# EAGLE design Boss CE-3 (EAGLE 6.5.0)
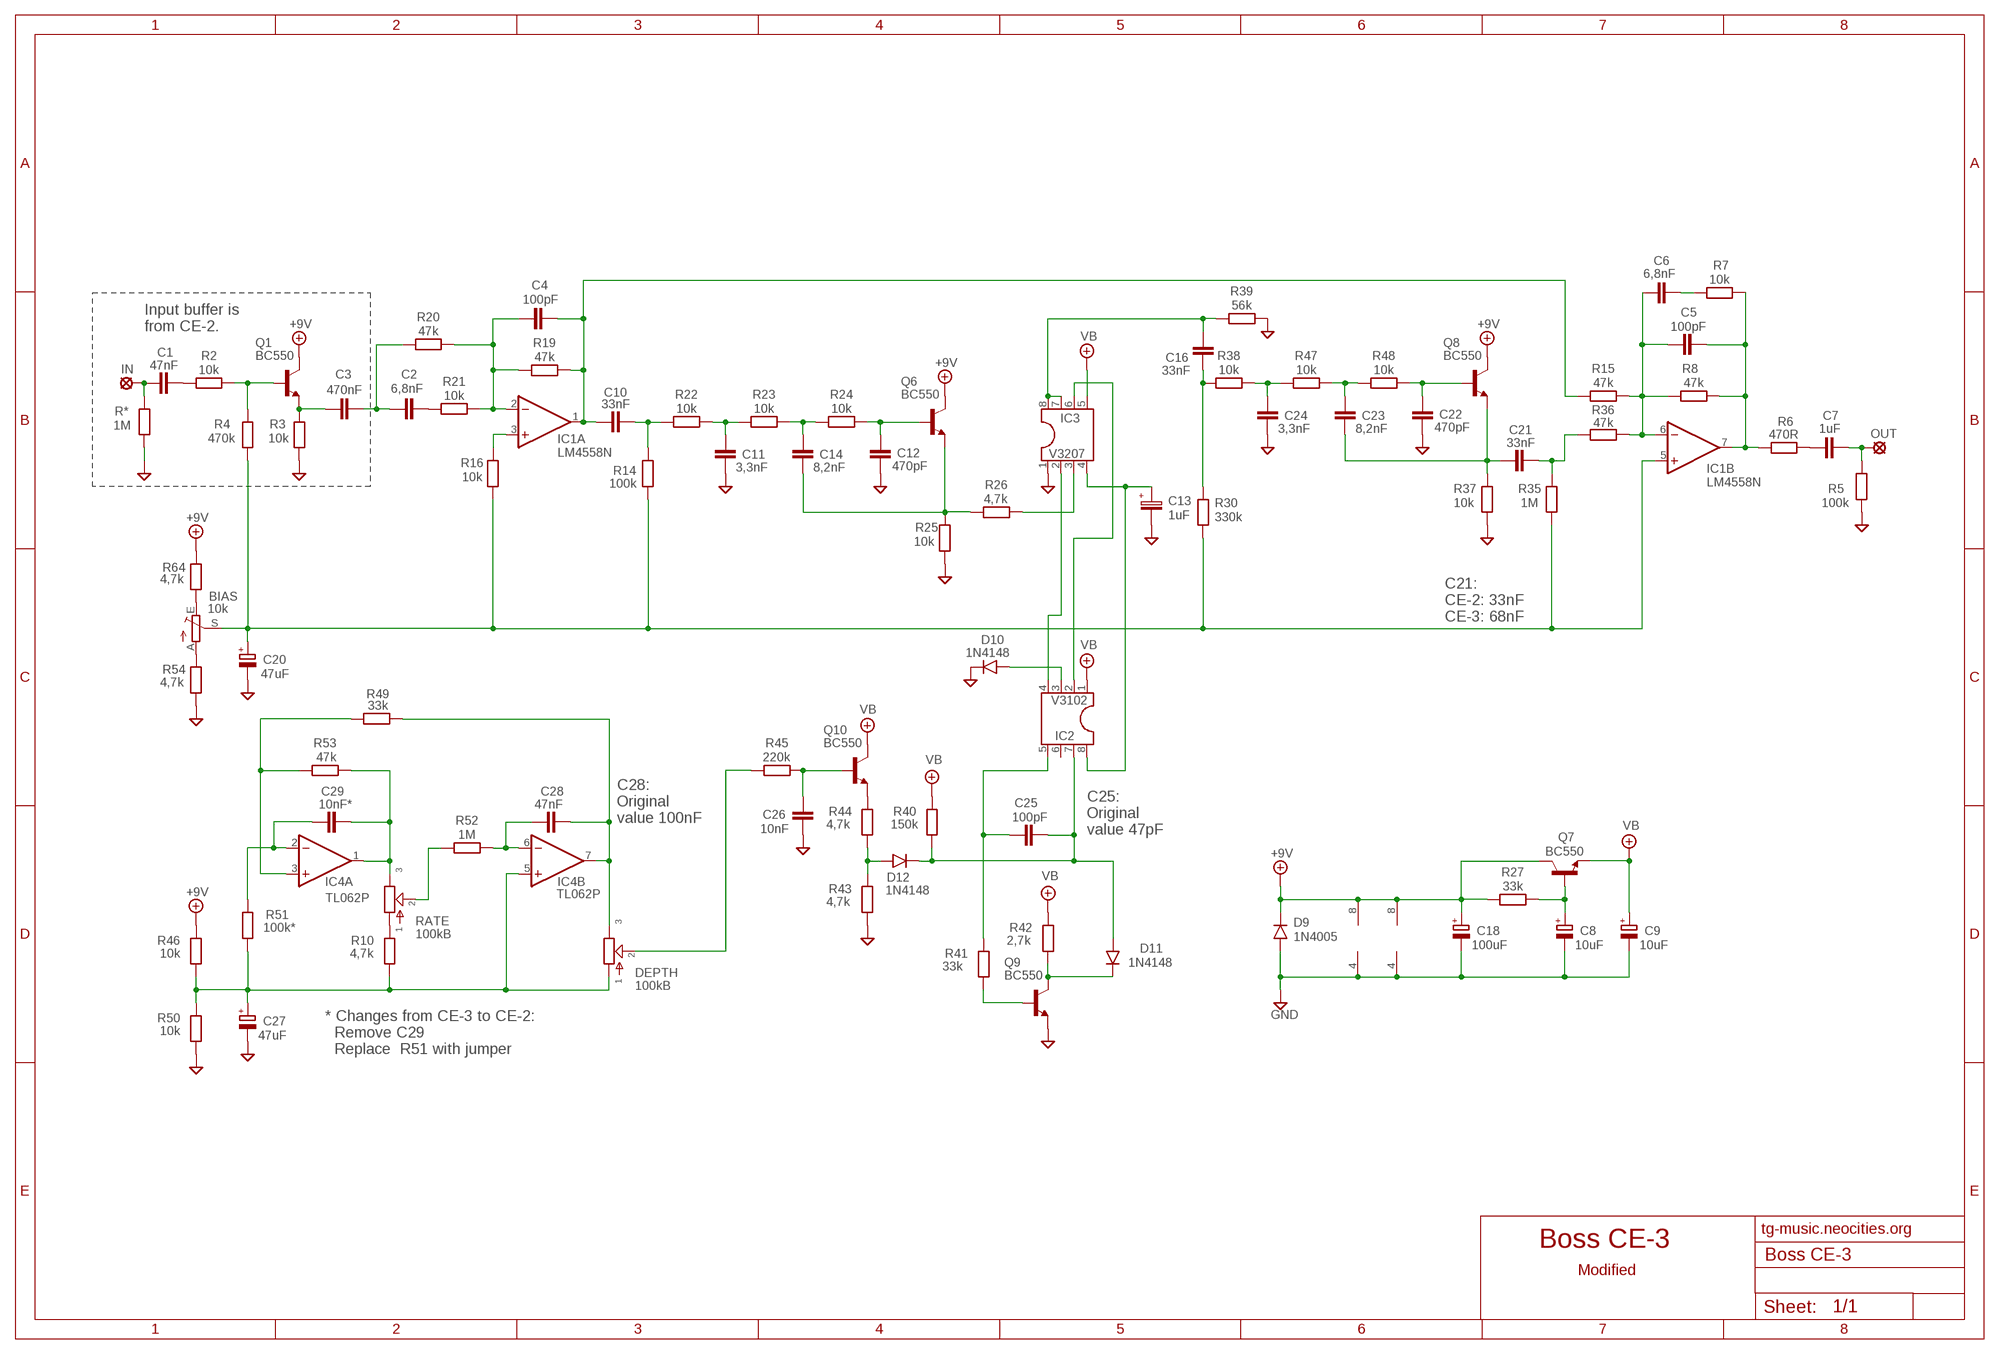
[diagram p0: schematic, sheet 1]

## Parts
+9V  +9V  +9V(T)1  [ROUND]
BIAS  10k  TRIM_EU-PT10  [PT-10]
C1  47nF  072X0252  [072X025]
C2  6,8nF  1NF-15NF  [3,5MM]
C3  470nF  072X0452  [072X045]
C4  100pF  050X030_0251  [050X030_025]
C5  100pF  050X030_0251  [050X030_025]
C6  6,8nF  1NF-15NF  [3,5MM]
C7  1uF  072X0352  [072X035]
C8  10uF  CPOL-EUB  [PANASONIC_B]
C9  10uF  CPOL-EUB  [PANASONIC_B]
C10  33nF  22NF-82NF"  [4,5MM]
C11  3,3nF  1NF-15NF  [3,5MM]
C12  470pF  050X030_0251  [050X030_025]
C13  1uF  050-EU  [050_020]
C14  8,2nF  1NF-15NF  [3,5MM]
C16  33nF  22NF-82NF"  [4,5MM]
C18  100uF  CPOL-EUD  [PANASONIC_D]
C20  47uF  CPOL-EUC  [PANASONIC_C]
C21  33nF  22NF-82NF"  [4,5MM]
C22  470pF  050X030_0251  [050X030_025]
C23  8,2nF  1NF-15NF  [3,5MM]
C24  3,3nF  1NF-15NF  [3,5MM]
C25  100pF  050X030_0251  [050X030_025]
C26  10nF  1NF-15NF  [3,5MM]
C27  47uF  CPOL-EUC  [PANASONIC_C]
C28  47nF  072X0252  [072X025]
C29  10nF*  1NF-15NF  [3,5MM]
D9  1N4005  1N400X.3  [DO41-3]
D10  1N4148  1N4148-3  [DO35-3]
D11  1N4148  1N4148-3  [DO35-3]
D12  1N4148  1N4148-3  [DO35-3]
DEPTH  100kB  POT-EU16MM  [16MM]
GND  GND  GND(T)1  [ROUND]
GND21  GND  GND(T)1  [ROUND]
IC1  LM4558N  [DIL08]
IC2  V3102  DIL8S  [SOCKET-08]
IC3  V3207  DIL8S  [SOCKET-08]
IC4  TL062P  [DIL08]
IN  MCS10B  [MCS10B]
OUT  MCS10B  [MCS10B]
Q1  BC550  [TO92-]
Q6  BC550  [TO92-]
Q7  BC550  [TO92-]
Q8  BC550  [TO92-]
Q9  BC550  [TO92-]
Q10  BC550  [TO92-]
R2  10k  6MM-EU1  [R0207/1V]
R3  10k  6MM-EU1  [R0207/1V]
R4  470k  6MM-EU1  [R0207/1V]
R5  100k  6MM-EU1  [R0207/1V]
R6  470R  6MM-EU1  [R0207/1V]
R7  10k  6MM-EU1  [R0207/1V]
R8  47k  6MM-EU1  [R0207/1V]
R10  4,7k  6MM-EU1  [R0207/1V]
R14  100k  6MM-EU1  [R0207/1V]
R15  47k  6MM-EU1  [R0207/1V]
R16  10k  6MM-EU1  [R0207/1V]
R19  47k  6MM-EU1  [R0207/1V]
R20  47k  6MM-EU1  [R0207/1V]
R21  10k  6MM-EU1  [R0207/1V]
R22  10k  6MM-EU1  [R0207/1V]
R23  10k  6MM-EU1  [R0207/1V]
R24  10k  6MM-EU1  [R0207/1V]
R25  10k  6MM-EU1  [R0207/1V]
R26  4,7k  6MM-EU1  [R0207/1V]
R27  33k  6MM-EU1  [R0207/1V]
R30  330k  6MM-EU1  [R0207/1V]
R35  1M  6MM-EU1  [R0207/1V]
R36  47k  6MM-EU1  [R0207/1V]
R37  10k  6MM-EU1  [R0207/1V]
R38  10k  6MM-EU1  [R0207/1V]
R39  56k  6MM-EU1  [R0207/1V]
R40  150k  6MM-EU1  [R0207/1V]
R41  33k  6MM-EU1  [R0207/1V]
R42  2,7k  6MM-EU1  [R0207/1V]
R43  4,7k  6MM-EU1  [R0207/1V]
R44  4,7k  6MM-EU1  [R0207/1V]
R45  220k  6MM-EU1  [R0207/1V]
R46  10k  6MM-EU1  [R0207/1V]
R47  10k  6MM-EU1  [R0207/1V]
R48  10k  6MM-EU1  [R0207/1V]
R49  33k  6MM-EU1  [R0207/1V]
R50  10k  6MM-EU1  [R0207/1V]
R51  100k*  6MM-EU1  [R0207/1V]
R52  1M  6MM-EU1  [R0207/1V]
R53  47k  6MM-EU1  [R0207/1V]
R54  4,7k  6MM-EU1  [R0207/1V]
R64  4,7k  6MM-EU1  [R0207/1V]
R*  1M  6MM-EU1  [R0207/1V]
RATE  100kB  POT-EU16MM  [16MM]

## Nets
+9V: +9V.1(+9V) C18.+ D9.C IC1.8(P:V+) IC4.8(P:V+) Q1.3(C) Q6.3(C) Q7.3(C) Q8.3(C) R27.1 R46.2 R64.2
BIAS: BIAS.S C20.+ IC1.5(B:+IN) R4.1 R14.2 R16.1 R30.1 R35.1
GND: C8.- C9.- C11.2 C12.1 C13.- C18.- C20.- C22.1 C24.2 C26.2 C27.- D9.A D10.C GND21.1(GND) GND.1(GND) IC1.4(P:V-) IC3.1 IC4.4(P:V-) Q9.1(E) R3.1 R5.2 R25.1 R37.1 R39.2 R43.1 R50.1 R54.1 R*.2
N$1: C1.2 R2.1
N$2: C1.1 IN.MP R*.1
N$3: C3.1 Q1.1(E) R3.2
N$4: Q1.2(B) R2.2 R4.2
N$5: C2.1 C3.2 R20.1
N$6: C2.2 R21.1
N$7: C4.1 IC1.2(A:-IN) R19.1 R20.2 R21.2
N$8: IC1.3(A:+IN) R16.2
N$9: C4.2 C10.1 IC1.1(A:OUT) R15.1 R19.2
N$10: C10.2 R14.1 R22.1
N$11: C11.1 R22.2 R23.1
N$12: C14.1 R23.2 R24.1
N$13: C12.2 Q6.2(B) R24.2
N$14: C14.2 Q6.1(E) R25.2 R26.2
N$15: IC3.3 R26.1
N$16: C16.2 IC3.7 IC3.8 R39.1
N$17: C13.+ IC2.8 IC3.4
N$18: C24.1 R38.2 R47.1
N$19: C23.1 R47.2 R48.1
N$20: C22.2 Q8.2(B) R48.2
N$21: C21.1 C23.2 Q8.1(E) R37.2
N$22: C21.2 R35.2 R36.1
N$23: C16.1 R30.2 R38.1
N$24: C5.1 C6.1 IC1.6(B:-IN) R8.1 R15.2 R36.2
N$25: C5.2 IC1.7(B:OUT) R6.2 R7.2 R8.2
N$26: C6.2 R7.1
N$27: C7.1 R6.1
N$28: C7.2 OUT.MP R5.1
N$29: D10.A IC2.3
N$30: IC2.2 IC3.6
N$31: IC2.4 IC3.2
N$32: C25.1 IC2.5 R41.2
N$33: C25.2 D11.A D12.C IC2.7 R40.1
N$34: D11.C Q9.3(C) R42.1
N$35: Q9.2(B) R41.1
N$36: D12.A R43.2 R44.1
N$37: Q10.1(E) R44.2
N$38: C26.1 Q10.2(B) R45.2
N$39: C28.2 DEPTH.3 IC4.7(B:OUT) R49.1
N$40: C28.1 IC4.6(B:-IN) R52.2
N$41: IC4.3(A:+IN) R49.2 R53.1
N$42: R10.2 RATE.1
N$43: R52.1 RATE.2
N$44: C29.2 IC4.1(A:OUT) R53.2 RATE.3
N$45: DEPTH.2 R45.1
N$46: C27.+ DEPTH.1 IC4.5(B:+IN) R10.1 R46.1 R50.2 R51.1
N$47: C29.1 IC4.2(A:-IN) R51.2
N$49: BIAS.E R64.1
N$50: BIAS.A R54.2
N$51: C8.+ Q7.2(B) R27.2
VB: C9.+ IC2.1 IC3.5 Q7.1(E) Q10.3(C) R40.2 R42.2
Unconnected: IC2.6

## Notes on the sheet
- Input buffer is
  from CE-2.
- C21:
  CE-2: 33nF
  CE-3: 68nF
- C28:
  Original 
  value 100nF
- C25:
  Original 
  value 47pF
- * Changes from CE-3 to CE-2:
    Remove C29
    Replace  R51 with jumper
- tg-music.neocities.org
- Boss CE-3
- Modified

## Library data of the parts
+9V = Virransyöttö:+9V(T): +9V Voltage Supply
BIAS = pot:TRIM_EU-: POTENTIOMETER
C1 C28 = Wima MKS:072X025: 1000pF - 0.47uF
C2 C6 C11 C14 C23 C24 C26 C29 = Mylar Kondensaattorit:1NF-15NF: 1nF-15nF
C3 = Wima MKS:072X045: 1.5uF
C4 C5 C12 C22 C25 = Keraamiset kondensaattorit:050X030_025: 47 - 120pF
C7 = Wima MKS:072X035: 0.15 - 1.0uF;
C8 C9 C18 C20 C27 = rcl:CPOL-EU: POLARIZED CAPACITOR, European symbol
C10 C16 C21 = Mylar Kondensaattorit:22NF-82NF: 22nF-82nF
C13 = Elektrolyytit:050-EU
D9 = Diodit:1N400X: Rectifier Diodes
D10-D12 = Diodit:1N4148: Fast Switching Diode
DEPTH RATE = potentiometers:POT-EU
GND GND21 = Virransyöttö:GND(T): Ground
IC1 = Operaatiovahvistimet:*4558: *4558 Op Amp Infamous for its use in tube screamers. This op amp has many manufacturers, hence the leading "*" in the name. The JRC4558 is a widely used example.
IC2 IC3 = ic-package:DIL8: Dual In Line / Socket
IC4 = Operaatiovahvistimet:TL062: OP AMP
IN OUT = Padit:MCS10B: SOLDER PAD
Q1 Q6-Q10 = Transistorit:BC550
R2-R8 R10 R14-R16 R19-R27 R30 R35-R54 R64 R* = vastukset:6MM-EU: 6mm Resistors (European schematic symbol)

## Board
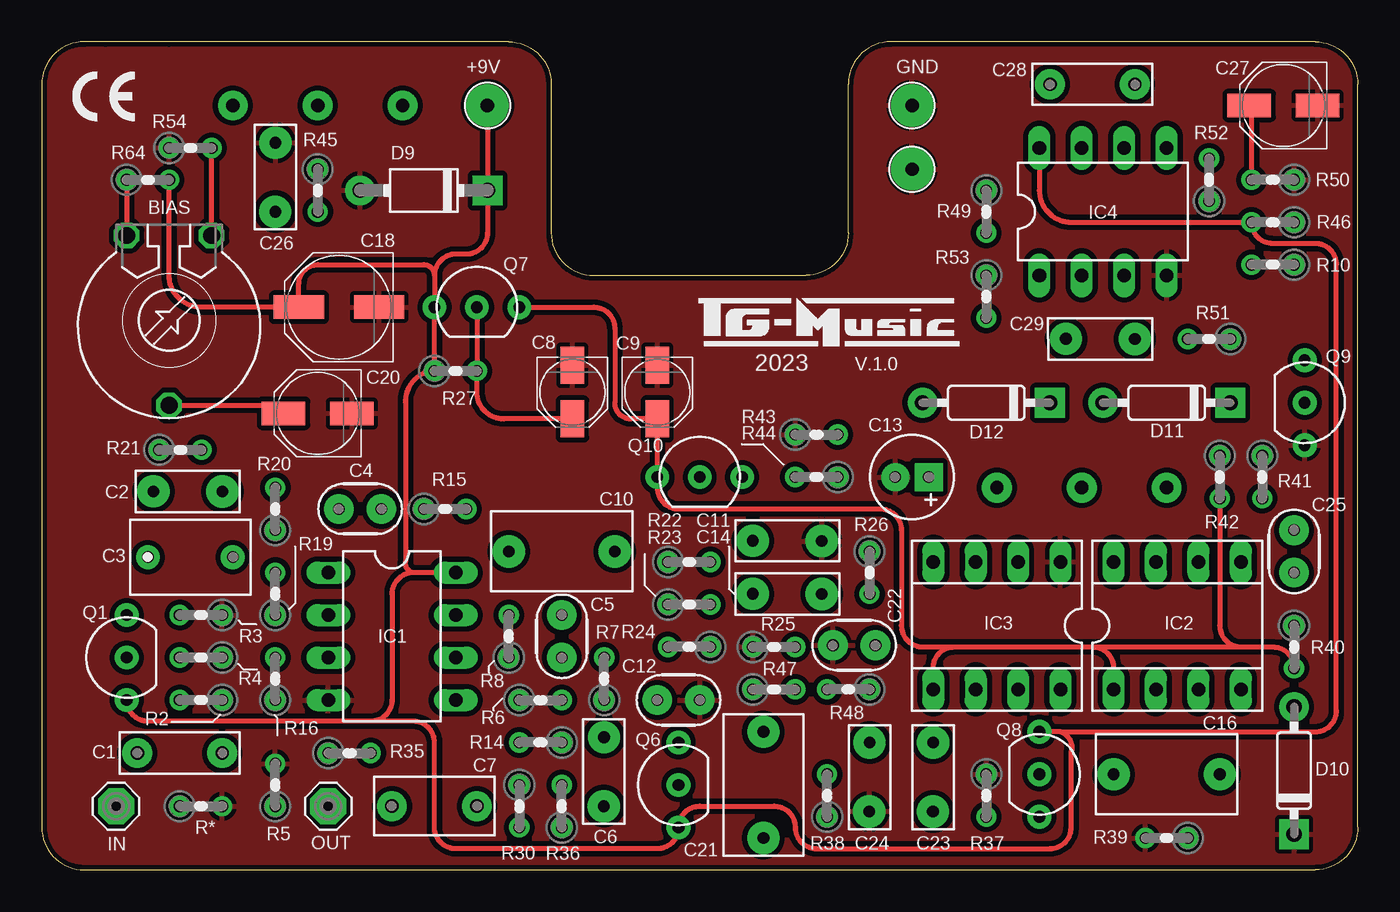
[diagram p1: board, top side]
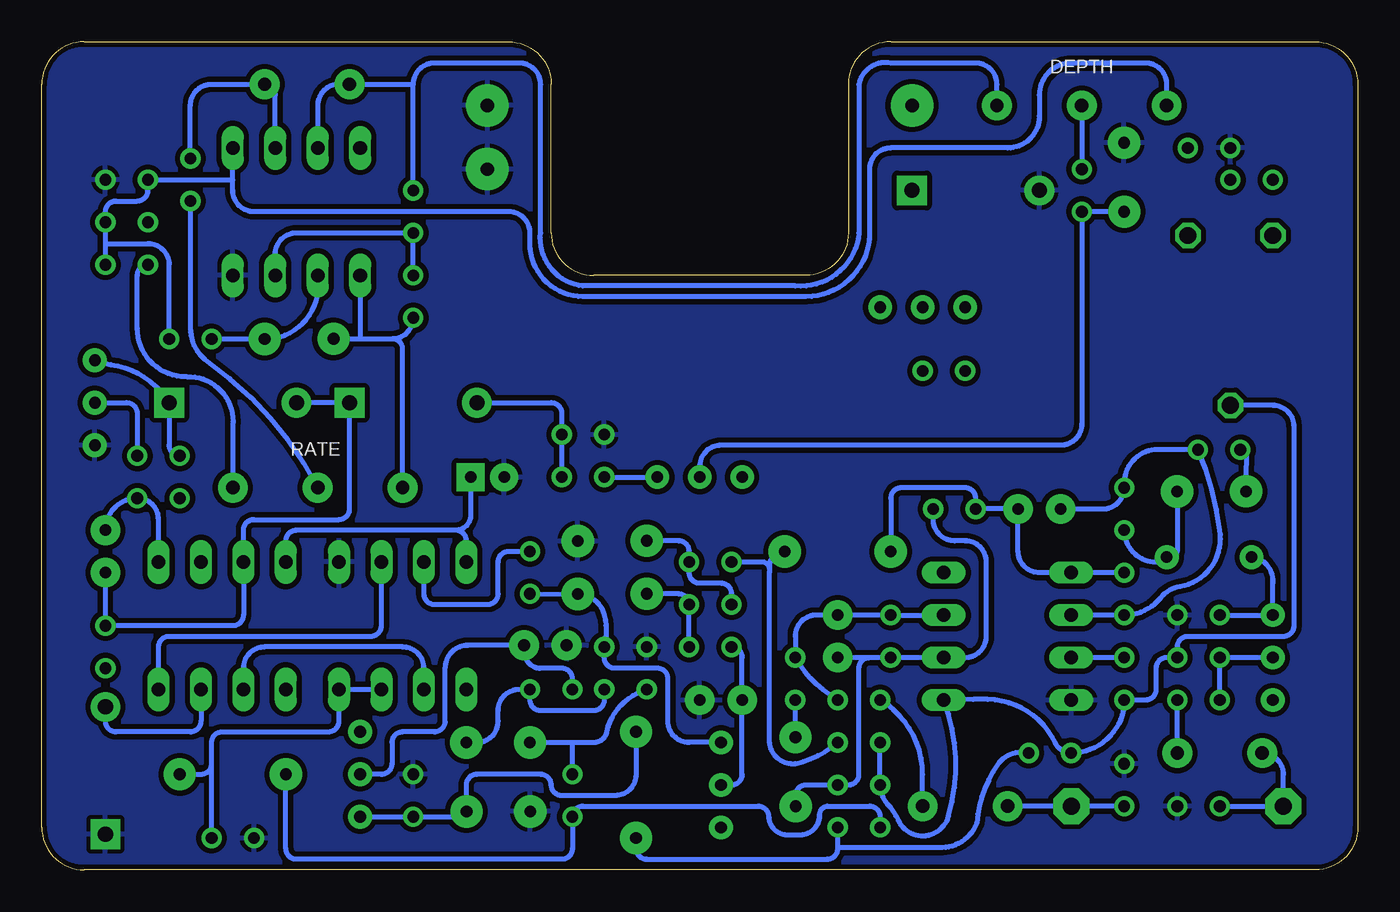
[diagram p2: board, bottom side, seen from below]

Size 78.74 x 49.53 mm. Coordinates in mm from the lower left corner, seen from the top.
Outline: 7.62,49.53 3.81,49.53
Outline: 78.74,2.54 78.74,46.99 arc90 76.2,49.53 50.8,49.53 arc90 48.26,46.99 48.26,38.1 arc-90 45.72,35.56 33.02,35.56 arc-90 30.48,38.1 30.48,46.99 arc90 27.94,49.53 2.54,49.53 arc90 0,46.99 0,2.54 arc90 2.54,0 76.2,0 arc90 78.74,2.54
Copper layers (1*16): Top 0.035mm / dielectric 1.5mm / Bottom 0.035mm
Design rules "ITEADstudio": minimum track width 10mil, minimum drill 12mil, track to track 12mil, track to pad 12mil, pad to pad 12mil, via to via 12mil, smd to smd 0mil, copper to edge 12mil, drill to drill 12mil, minimum pad ring 10mil, minimum via ring 6mil, stop-mask expansion 4mil, vias tented up to drill 100mil, thermal gap 10mil

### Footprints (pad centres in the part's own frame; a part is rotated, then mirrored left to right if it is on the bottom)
ROUND = drill 0.8 pad 2.54: 1 0,0
PT-10 = drill 1.016 octagon: A -2.54,-5.08; E 2.54,-5.08; S 0,5.08
072X025 = drill 0.8 pad 1.778: 1 -2.54,0; 2 2.54,0
3,5MM = drill 0.7 pad 1.93: 1 -1.905,0; 2 2.221,-0.016
072X045 = drill 0.7 pad 1.422: 1 -2.54,0; 2 2.54,0
050X030_025 = drill 0.7 pad 1.778: 1 -1.27,0; 2 1.27,0
072X035 = drill 0.8 pad 1.778: 1 -2.54,0; 2 2.54,0
PANASONIC_B = smd 2.2 x 1.4: + 1.6,0; - -1.6,0
4,5MM = drill 0.7 pad 1.93: 1 -3.175,0; 2 3.175,0
050_020 = drill 0.7 pad 1.676 square: + -1,0 | drill 0.7 pad 1.676: - 1,0
PANASONIC_D = smd 3 x 1.4: + 2.4,0; - -2.4,0
PANASONIC_C = smd 2.6 x 1.4: + 2.05,0; - -2.05,0
DO41-3 = drill 0.9 pad 1.778: A 3.81,0 | drill 0.9 pad 1.778 square: C -3.81,0
DO35-3 = drill 0.9 pad 1.778: A 3.81,0 | drill 0.9 pad 1.778 square: C -3.81,0
16MM = drill 0.8 pad 1.778: 1 5.08,0; 2 0,0; 3 -5.08,0
DIL08 = drill 0.813 long: 1 -3.81,-3.81; 2 -1.27,-3.81; 3 1.27,-3.81; 4 3.81,-3.81; 5 3.81,3.81; 6 1.27,3.81; 7 -1.27,3.81; 8 -3.81,3.81
SOCKET-08 = drill 0.813 long: 1 -3.81,-3.81; 2 -1.27,-3.81; 3 1.27,-3.81; 4 3.81,-3.81; 5 3.81,3.81; 6 1.27,3.81; 7 -1.27,3.81; 8 -3.81,3.81
MCS10B = drill 1.016 pad 2.159 octagon: MP 0,0
TO92- = drill 0.7 pad 1.422: 1 2.54,0; 2 0,0; 3 -2.54,0
R0207/1V = drill 0.7: 1 -1.27,0; 2 1.27,0

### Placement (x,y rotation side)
+9V  26.67,45.72 0 top
BIAS  7.62,32.86 180 top
C1  8.26,6.99 0 top
C2  8.9,22.62 180 top
C3  8.89,18.71 0 top
C4  19.05,21.59 0 top
C5  31.11,13.97 90 top
C6  33.62,5.71 90 top
C7  23.5,3.81 180 top
C8  31.75,28.57 270 top
C9  36.83,28.57 270 top
C10  31.11,19.05 0 top
C11  44.45,19.68 0 top
C12  38.1,10.16 180 top
C13  52.07,23.5 180 top
C14  44.45,16.51 0 top
C16  67.31,5.71 0 top
C18  17.78,33.66 180 top
C20  16.51,27.3 180 top
C21  43.18,5.08 270 top
C22  48.61,13.43 0 top
C23  53.34,5.71 270 top
C24  49.53,5.71 270 top
C25  74.93,19.05 270 top
C26  13.97,41.27 90 top
C27  74.3,45.72 180 top
C28  62.87,46.99 180 top
C29  63.5,31.75 180 top
D9  22.86,40.64 180 top
D10  74.93,5.94 90 top
D11  67.31,27.94 180 top
D12  56.52,27.94 180 top
DEPTH  16.51,45.72 0 bottom
GND  52.07,45.72 0 top
GND21  52.07,41.91 0 top
IC1  20.95,13.97 270 top
IC2  67.94,14.61 0 top
IC3  57.15,14.61 180 top
IC4  63.5,39.37 0 top
IN  4.45,3.81 0 top
OUT  17.14,3.81 0 top
Q1  5.08,12.7 90 top
Q6  38.1,5.08 90 top
Q7  26.04,33.66 0 top
Q8  59.69,5.71 270 top
Q9  75.56,27.94 270 top
Q10  39.37,23.5 0 top
R2  9.53,10.16 180 top
R3  9.53,15.24 180 top
R4  9.53,12.7 180 top
R5  13.97,5.08 90 top
R6  29.84,10.16 0 top
R7  33.66,11.43 90 top
R8  27.94,13.97 90 top
R10  73.66,36.2 180 top
R14  29.84,7.62 180 top
R15  24.13,21.59 0 top
R16  13.97,11.43 90 top
R19  13.97,16.51 90 top
R20  13.97,21.59 90 top
R21  8.29,25.13 0 top
R22  38.73,18.41 0 top
R23  38.73,15.88 0 top
R24  38.73,13.34 180 top
R25  43.81,13.34 0 top
R26  49.53,17.78 270 top
R27  24.77,29.84 0 top
R30  28.57,3.81 270 top
R35  18.41,6.99 0 top
R36  31.11,3.81 90 top
R37  56.52,4.45 270 top
R38  46.99,4.45 90 top
R39  67.31,1.91 180 top
R40  74.93,13.34 270 top
R41  73.03,23.5 270 top
R42  70.48,23.5 270 top
R43  46.35,26.04 0 top
R44  46.35,23.5 180 top
R45  16.51,40.64 270 top
R46  73.66,38.73 180 top
R47  43.81,10.79 0 top
R48  48.26,10.79 180 top
R49  56.52,39.37 270 top
R50  73.66,41.27 180 top
R51  69.85,31.75 180 top
R52  69.85,41.27 90 top
R53  56.52,34.29 270 top
R54  8.89,43.18 0 top
R64  6.35,41.27 0 top
R*  9.53,3.81 0 top
RATE  62.23,22.86 180 bottom

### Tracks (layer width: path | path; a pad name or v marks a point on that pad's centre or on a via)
+9V
  Top 0.305: +9V.1 D9.C 26.67,38.1 arc-90 25.4,36.83 24.77,36.83 arc90 23.5,35.56 | 23.5,35.56 Q7.3 R27.1 arc90 21.76,27.94 21.76,18.41 arc90 22.23,17.78 | R64.2 7.62,35.56 arc90 9.53,33.66 C18.+ 15.38,35.06 arc-90 16.51,36.2 22.86,36.2 arc-90 23.5,35.56 | IC4.8 59.69,40.64 arc90 61.59,38.73 R46.2 arc90 73.66,37.47 76.2,37.47 arc-90 77.47,36.2 77.47,9.53 arc-90 76.2,8.26 60.96,8.26 | IC1.8 22.23,17.78 | 22.23,17.78 arc90 20.95,16.51 20.95,10.16 arc-90 19.68,8.89 | 19.68,8.89 6.35,8.89 arc-90 Q1.3 | 19.68,8.89 22.23,8.89 arc-90 23.5,7.62 23.5,2.54 arc90 24.77,1.27 36.83,1.27 arc90 Q6.3 arc-90 39.37,3.81 43.81,3.81 arc-90 45.09,2.54 arc90 46.35,1.27 60.33,1.27 arc90 61.59,2.54 61.59,6.99 arc90 60.96,8.26 | 60.96,8.26 Q8.3
BIAS
  Top 0.305: BIAS.S 11.45,27.78 13.98,27.78 arc-90 C20.+
  Bottom 0.305: BIAS.S 5.08,27.78 arc90 3.81,26.51 3.81,14.61 arc90 4.45,13.97 10.16,13.97 arc-90 10.79,13.34 R4.1 11.43,12.7 arc-90 12.06,12.06 12.06,10.79 arc90 12.7,10.16 R16.1 arc90 R35.1 arc65 18.1,7.59 arc-64 22.13,10.19 arc-3 IC1.5 arc37 24.48,3.21 arc138 27.5,2.95 arc-15 28.16,3.97 arc41 R30.1 R14.2
GND
  pour Bottom: 0,2.54 0,46.99 arc-90 2.54,49.53 27.94,49.53 arc-90 30.48,46.99 30.48,38.1 arc90 33.02,35.56 45.72,35.56 arc90 48.26,38.1 48.26,46.99 arc-90 50.8,49.53 76.2,49.53 arc-90 78.74,46.99 78.74,2.54 arc-90 76.2,0 2.54,0 arc-90
  pour Top: 0,2.54 0,46.99 arc-90 2.54,49.53 27.94,49.53 arc-90 30.48,46.99 30.48,38.1 arc90 33.02,35.56 45.72,35.56 arc90 48.26,38.1 48.26,46.99 arc-90 50.8,49.53 76.2,49.53 arc-90 78.74,46.99 78.74,2.54 arc-90 76.2,0 2.54,0 arc-90
N$1
  Bottom 0.305: C1.2 R2.1
N$2
  Bottom 0.305: R*.1 IN.MP 4.45,5.71 arc-90 C1.1
N$3
  Bottom 0.305: R3.2 Q1.1 5.08,17.14 arc-90 C3.1
N$4
  Bottom 0.305: Q1.2 R4.2 R2.2
N$5
  Bottom 0.305: C2.1 10.79,19.05 arc90 C3.2 12.06,18.41 arc90 R20.1
N$6
  Bottom 0.305: C2.2 6.64,24.73 arc-90 R21.1
N$7
  Bottom 0.305: IC1.2 R19.1 arc-51 11.78,16.29 arc42 10.64,16.95 arc-91 8.26,20.32 arc-17 R21.2 12.15,25.14 arc-90 R20.2 arc90 15.24,21.59 C4.1
N$8
  Bottom 0.305: R16.2 IC1.3
N$9
  Bottom 0.305: R19.2 IC1.1 19.05,17.78 arc90 20.32,19.05 C4.2 R15.1 22.86,22.23 arc-90 23.5,22.86 27.3,22.86 arc-90 27.94,22.23 C10.1
N$10
  Bottom 0.305: 35.21,17.78 35.21,7.62 arc-90 33.66,6.35 arc-28 R14.1 | R22.1 35.56,18.41 arc90 35.21,17.78 | C10.2 arc-90 35.21,18.13 35.21,17.78
N$11
  Bottom 0.305: R23.1 37.47,16.51 arc-90 38.1,17.14 39.37,17.14 arc90 40.01,17.78 R22.2 40.01,19.05 arc-90 40.64,19.68 C11.1
N$12
  Bottom 0.305: R24.1 R23.2 arc-90 40.64,16.51 C14.1
N$13
  Bottom 0.305: Q6.2 37.47,5.08 arc-90 36.83,5.71 C12.2 36.83,12.7 arc-90 R24.2
N$14
  Bottom 0.305: Q6.1 40.01,7.62 arc90 41.27,8.89 41.27,11.43 arc-90 41.91,12.06 44.45,12.06 arc90 45.09,12.68 R25.2 arc-27 45.09,15.24 arc-76 C14.2 R26.2
N$15
  Bottom 0.305: IC3.3 55.88,16.51 arc-90 55.24,15.88 52.07,15.88 arc-90 51.44,16.51 51.44,18.41 arc90 50.8,19.05 R26.1
N$16
  Bottom 0.305: IC3.7 IC3.8 60.96,8.89 arc90 61.59,8.26 67.94,8.26 arc-90 68.58,7.62 68.58,6.35 | C16.2 69.22,5.71 arc-90 68.58,6.35 | R39.1 68.58,6.35
N$17
  Bottom 0.305: IC2.8 64.14,19.68 arc90 63.5,20.32 53.98,20.32 | IC3.4 53.34,19.68 arc-90 53.98,20.32 | C13.+ 53.07,21.23 arc90 53.98,20.32
N$18
  Bottom 0.305: C24.1 46.99,7.62 | 46.99,7.62 45.72,7.62 arc-77 44.93,8.26 arc61 R47.1 | R38.2 46.99,7.62
N$19
  Bottom 0.305: C23.1 52.7,7.62 arc-90 51.44,8.89 51.44,9.53 arc90 50.16,10.79 R48.1 49.53,10.16 arc-90 48.9,9.53 45.72,9.53 arc-90 45.09,10.16 R47.2
N$20
  Bottom 0.305: Q8.2 58.42,5.71 arc-90 57.78,6.35 57.78,7.62 arc90 57.15,8.26 55.24,8.26 arc-90 54.61,8.89 54.61,12.06 arc90 53.24,13.43 C22.2 49.88,13.05 arc-90 48.9,12.06 47.62,12.06 arc90 46.99,11.43 R48.2
N$21
  Bottom 0.305: C21.1 43.18,5.71 arc90 44.45,4.45 47.62,4.45 arc90 48.26,5.08 arc-90 48.9,5.71 52.7,5.71 arc-90 53.34,5.08 53.34,3.51 arc-90 C23.2 arc90 53.64,3.17 R37.2 Q8.1
N$22
  Bottom 0.305: C21.2 43.18,1.27 arc-90 42.55,0.64 31.75,0.64 arc-90 31.11,1.27 31.11,1.33 | 31.11,1.33 R36.1 | 31.11,1.33 25.08,1.33 arc-73 22.8,2.79 arc31 21.53,6.32 arc69 R35.2
N$23
  Bottom 0.305: C16.1 64.14,1.27 arc-90 63.5,0.64 47.62,0.64 arc-90 46.99,1.27 R38.1 arc90 46.35,3.81 35.88,3.81 arc90 35.24,3.17 arc-90 34.07,2.1 33.43,2.1 arc-90 32.19,3.21 arc90 31.75,3.81 29.21,3.81 arc90 28.57,3.17 R30.2
N$24
  Bottom 0.305: R15.2 25.4,20.95 arc-90 24.13,19.68 23.5,19.68 arc90 22.23,18.41 22.23,13.97 arc90 23.5,12.7 IC1.6 R8.1 29.21,12.7 | 29.21,12.7 C5.1 | C6.1 33.62,4.48 arc90 33.02,5.08 R36.2 30.48,5.08 arc-90 29.84,5.71 29.84,12.06 arc90 29.21,12.7
N$25
  Bottom 0.305: IC1.7 R8.2 C5.2 32.38,15.24 arc-90 33.66,13.97 R7.2 arc-27 31.59,10.48 R6.2
N$26
  Bottom 0.305: C6.2 R7.1
N$27
  Bottom 0.305: C7.1 26.04,5.71 arc-59 R6.1
N$28
  Bottom 0.305: R5.1 OUT.MP C7.2
N$29
  Bottom 0.305: IC2.3 69.22,8.89 arc90 69.85,8.26 74.3,8.26 arc90 74.93,8.89 D10.A
N$30
  Bottom 0.305: IC3.6 55.88,12.06 arc-90 57.15,13.34 65.41,13.34 arc-90 66.67,12.06 IC2.2
N$31
  Bottom 0.305: IC2.4 71.75,13.34 arc90 71.12,13.97 59.05,13.97 arc-90 58.42,14.61 IC3.2
N$32
  Bottom 0.305: C25.1 arc90 R41.2 arc90 71.75,20.95 IC2.5
N$33
  Bottom 0.305: C25.2 R40.1 67.31,14.61 arc-90 66.67,15.24 IC2.7 66.67,20.32 arc90 66.04,20.95 60.96,20.95 arc-90 60.33,21.59 D12.C D11.A
N$34
  Bottom 0.305: R42.1 arc90 71.12,25.4 D11.C arc-50 74.61,30.23 Q9.3
N$35
  Bottom 0.305: Q9.2 73.66,27.94 arc90 73.03,27.3 R41.1
N$36
  Bottom 0.305: D12.A 48.26,27.94 arc90 47.62,27.3 R43.2 R44.1
N$37
  Bottom 0.305: R44.2 Q10.1
N$38
  Bottom 0.305: C26.1 R45.2 16.51,26.67 arc90 17.78,25.4 38.1,25.4 arc-90 39.37,24.13 Q10.2
N$39
  Bottom 0.305: DEPTH.3 21.59,46.99 arc-90 22.86,48.26 27.94,48.26 arc-90 29.84,46.99 29.84,38.1 arc90 33.66,34.92 46.35,34.92 arc90 48.9,38.1 48.9,46.99 arc-90 50.16,48.26 55.24,48.26 arc-90 56.52,46.99 | 56.52,46.99 C28.2 60.96,46.99 arc-90 62.23,45.72 IC4.7 | R49.1 56.52,46.99
N$40
  Bottom 0.305: IC4.6 64.77,46.35 arc-90 C28.1 68.58,46.99 arc-90 69.85,45.72 R52.2
N$41
  Bottom 0.305: IC4.3 64.77,36.83 arc90 63.5,38.1 R49.2 R53.1
N$42
  Bottom 0.305: RATE.1 67.31,26.57 arc-98 70.07,29.5 70.14,29.5 arc90 73.03,32.38 73.03,35.56 arc90 R10.2
N$43
  Bottom 0.305: R52.1 69.85,32.38 arc-55 68.83,30.42 arc27 RATE.2
N$44
  Bottom 0.305: C29.2 59.69,31.77 | 59.69,31.77 57.77,31.77 | 57.77,31.77 arc-90 R53.2 | IC4.1 59.69,31.77 | RATE.3 57.15,31.15 arc-90 57.77,31.77
N$45
  Bottom 0.305: DEPTH.2 R45.1
N$46
  Top 0.305: R50.2 72.39,45.58 arc90 C27.+
  Bottom 0.305: DEPTH.1 11.43,46.99 arc-90 12.7,48.26 17.14,48.26 arc-90 19.05,46.35 19.05,45.09 arc90 20.95,43.18 27.94,43.18 arc-90 29.21,41.91 29.21,38.1 arc90 33.02,34.29 46.35,34.29 arc90 49.53,37.47 49.53,38.1 arc-90 50.8,39.37 66.04,39.37 arc90 67.31,40.64 67.31,41.27 | 67.31,41.27 IC4.5 | 67.31,41.27 R50.2 72.39,40.64 arc90 73.03,40.01 74.3,40.01 arc-90 74.93,39.37 R46.1 74.93,37.47 | 74.93,37.47 R10.1 | R51.1 71.12,36.2 arc-90 72.39,37.47 74.93,37.47
N$47
  Bottom 0.305: IC4.2 arc100 C29.1 R51.2
N$49
  Top 0.305: R64.1 BIAS.E
N$50
  Top 0.305: BIAS.A R54.2
N$51
  Top 0.305: Q7.2 R27.2 26.04,28.57 arc90 27.64,26.98 C8.+
VB
  Top 0.305: Q7.1 33.02,33.66 arc-90 34.29,32.38 34.29,27.94 arc90 35.26,26.98 C9.+ Q10.3 36.83,22.86 arc90 38.1,21.59 50.16,21.59 arc-90 51.44,20.32 51.44,14.61 arc90 52.7,13.34 54.61,13.34 | R42.2 70.48,14.61 arc90 71.75,13.34 | 71.75,13.34 73.66,13.34 arc-90 R40.2 | IC3.5 53.34,12.06 arc-90 54.61,13.34 | 54.61,13.34 62.87,13.34 | 62.87,13.34 arc-90 64.14,12.06 IC2.1 | 62.87,13.34 71.75,13.34

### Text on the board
tNames: 2023 | V.1.0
